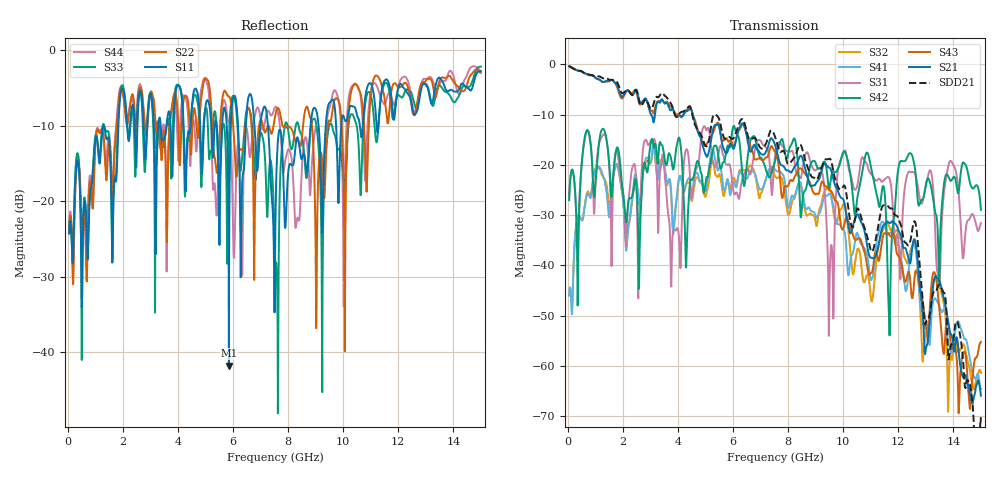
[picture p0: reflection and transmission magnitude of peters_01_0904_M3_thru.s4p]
# MHZ S RI R 50.00
! FREQ  S11  S12  S13  S14
!  S21  S22  S23  S24
!  S31  S32  S33  S34
!  S41  S42  S43  S44
!  REAL  IMAG  REAL  IMAG  REAL  IMAG  REAL  IMAG
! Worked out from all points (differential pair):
!   1496 points, 50 MHz to 15 GHz, reference 50 ohm
!   strongest paths, dB at 50 MHz, 3.79 GHz, 7.53 GHz, 11.27 GHz, 15 GHz:
!     S21: -0.4, -8.9, -16.0, -36.3, -66.0
!     S43: -0.4, -8.6, -17.4, -38.9, -55.2
!     S42: -27.0, -20.0, -19.2, -27.3, -28.9
!     S31: -27.0, -35.7, -18.1, -22.8, -31.6
!     S41: -46.0, -29.4, -20.9, -33.8, -64.6
!     S32: -46.0, -30.4, -22.3, -36.7, -61.4
!   taken as a pair (ports 1,3 in; 2,4 out), SDD21 dB: -0.3, -8.3, -14.4, -32.3, -70.2
!   lowest |S11| = -41.8 dB at 5.85 GHz (marker M1), VSWR 1.02, Z = 50.5 - j0.674 ohm
!   |S11| at or under -10 dB: start of sweep to 1.839 GHz; 6.183 GHz to 6.471 GHz (288.1 MHz wide, 4.55 % of centre); 7.267 GHz to 8.817 GHz (1.55 GHz wide, 19.3 % of centre)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
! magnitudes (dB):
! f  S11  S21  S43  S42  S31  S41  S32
! 50 MHz  -24.3  -0.4  -0.4  -27.0  -27.0  -46.0  -46.0
! 5.85 GHz  -41.8  -16.5  -15.4  -16.5  -19.9  -24.0  -24.3
! 9.5 GHz  -7.0  -20.6  -25.1  -24.6  -45.6  -25.7  -24.5
! 10.88 GHz  -4.9  -36.5  -40.4  -17.6  -20.2  -38.2  -41.9
! 11.67 GHz  -4.5  -31.6  -33.8  -51.1  -22.5  -33.7  -32.2
! 12.1 GHz  -4.5  -34.2  -39.5  -19.2  -39.9  -38.5  -34.8
! 15 GHz  -2.8  -66.0  -55.2  -28.9  -31.6  -64.6  -61.4
